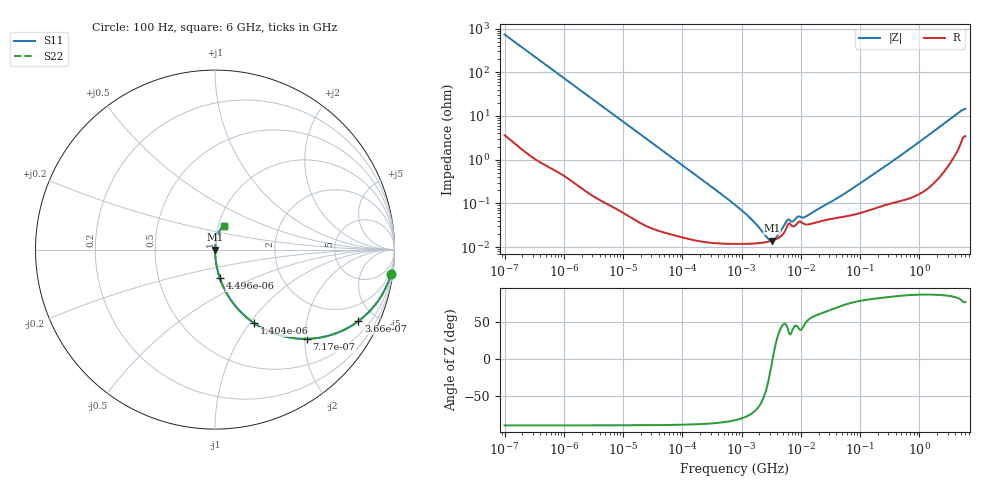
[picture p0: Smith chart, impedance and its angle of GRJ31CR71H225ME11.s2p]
!Murata Part Number: GRJ31CR71H225ME11
!These Parameters are Measured in Series Mode Connection
!Data Generated on Jun 19, 2026
!  o--ll--o
!Port1  Port2
!  o------o
!Operation Temp=25[degC], DC Bias Voltage=0[V]
!Freq. Start=100[Hz] Stop=6[GHz] 401[Steps]
# Hz S RI R 50
!Freq.(Hz) S11(Real) S11(Imag) S21(Real) S21(Imag) S12(Real) S12(Imag) S22(Real) S22(Imag)
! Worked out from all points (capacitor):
!   401 points, 100 Hz to 6 GHz, reference 50 ohm
!   read as one part in series: C = 2.18 uF near 109 Hz
!   lowest |Z| = 14.1 mohm at 3.246 MHz (marker M1)
!   series resonance near 3.35 MHz, so ESL is about 1 nH
!   S11 on the Smith chart (normalised r, x): 100 Hz: 1, -15; 366 Hz: 1.02, -4.00; 717 Hz: 1.01, -2.05; 1.404 kHz: 1.01, -1.05; 4.496 kHz: 1.00, -0.33; 6 GHz: 1.07, +0.28
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100  0.981 -0.1342  0.019 0.1342  0.019 0.1342  0.981 -0.1342
205  0.9265 -0.2587  0.0735 0.2587  0.0735 0.2587  0.9265 -0.2587
366  0.799 -0.3984  0.201 0.3984  0.201 0.3984  0.799 -0.3984
717  0.5119 -0.4971  0.4881 0.4971  0.4881 0.4971  0.5119 -0.4971
1404  0.2173 -0.4094  0.7827 0.4094  0.7827 0.4094  0.2173 -0.4094
2008  0.1203 -0.3223  0.8797 0.3223  0.8797 0.3223  0.1203 -0.3223
4496  0.0273 -0.1598  0.9727 0.1598  0.9727 0.1598  0.0273 -0.1598
11514  0.00468 -0.0642  0.9953 0.0642  0.9953 0.0642  0.00468 -0.0642
40335  0.000576 -0.0185  0.9994 0.0185  0.9994 0.0185  0.000576 -0.0185
774597  0.00012 -0.000923  0.9999 0.000923  0.9999 0.000923  0.00012 -0.000923
1516199  0.000121 -0.000398  0.9999 0.000398  0.9999 0.000398  0.000121 -0.000398
2713602  0.000132 -9.73e-05  0.9999 9.73e-05  0.9999 9.73e-05  0.000132 -9.73e-05
3245845  0.000141 -1.46e-05  0.9999 1.46e-05  0.9999 1.46e-05  0.000141 -1.46e-05
3882480  0.000154 6.96e-05  0.9998 -6.96e-05  0.9998 -6.96e-05  0.000154 6.96e-05
5809218  0.000289 0.00028  0.9997 -0.00028  0.9997 -0.00028  0.000289 0.00028
9090158  0.000375 0.000333  0.9996 -0.000333  0.9996 -0.000333  0.000375 0.000333
1.189169e7  0.000332 0.000364  0.9997 -0.000364  0.9997 -0.000364  0.000332 0.000364
1.555665e7  0.000346 0.000513  0.9997 -0.000513  0.9997 -0.000513  0.000346 0.000513
5.449875e7  0.0005 0.00159  0.9995 -0.00159  0.9995 -0.00159  0.0005 0.00159
3.124326e8  0.00104 0.00816  0.999 -0.00816  0.999 -0.00816  0.00104 0.00816
4.586474e9  0.0302 0.1118  0.9698 -0.1118  0.9698 -0.1118  0.0302 0.1118
6e9  0.0512 0.1298  0.9488 -0.1298  0.9488 -0.1298  0.0512 0.1298
